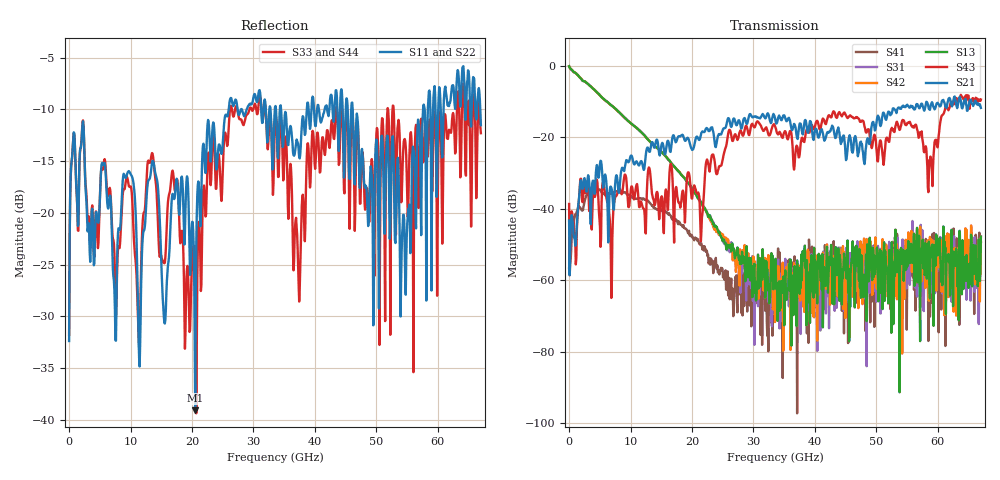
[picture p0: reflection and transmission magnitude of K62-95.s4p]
!Agilent Technologies,N5247A,US50470101,A.10.25.02
!Agilent N5247A: A.10.25.02
!Date: Tuesday, May 12, 2015 13:46:24
!Correction: Sdd11(Full 4 Port(1,2,3,4))
!Sdc11(Full 4 Port(1,2,3,4))
!Sdd12(Full 4 Port(1,2,3,4))
!Sdc12(Full 4 Port(1,2,3,4))
!Scd11(Full 4 Port(1,2,3,4))
!Scc11(Full 4 Port(1,2,3,4))
!Scd12(Full 4 Port(1,2,3,4))
!Scc12(Full 4 Port(1,2,3,4))
!Sdd21(Full 4 Port(1,2,3,4))
!Sdc21(Full 4 Port(1,2,3,4))
!Sdd22(Full 4 Port(1,2,3,4))
!Sdc22(Full 4 Port(1,2,3,4))
!Scd21(Full 4 Port(1,2,3,4))
!Scc21(Full 4 Port(1,2,3,4))
!Scd22(Full 4 Port(1,2,3,4))
!Scc22(Full 4 Port(1,2,3,4))
!Balanced Topology: BBAL
!S4P File: Measurements: <Sdd11,Sdc11,Sdd12,Sdc12>,
!<Scd11,Scc11,Scd12,Scc12>,
!<Sdd21,Sdc21,Sdd22,Sdc22>,
!<Scd21,Scc21,Scd22,Scc22>:
# Hz S  dB  R 50
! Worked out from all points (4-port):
!   801 points, 10 MHz to 67 GHz, reference 50 ohm
!   strongest paths, dB at 10 MHz, 16.76 GHz, 33.51 GHz, 50.25 GHz, 67 GHz:
!     S21: -43.3, -20.7, -14.6, -13.9, -11.8
!     S43: -38.6, -29.4, -16.9, -26.7, -9.4
!     S13: -0.1, -27.5, -55.4, -61.9, -47.8
!     S42: -0.1, -27.5, -71.7, -51.7, -49.3
!     S31: -0.1, -27.5, -60.2, -50.4, -49.3
!     S41: -56.7, -42.4, -57.1, -55.7, -47.8
!   lowest |S11| = -39.1 dB at 20.53 GHz (marker M1), VSWR 1.02, Z = 51 - j0.416 ohm
!   |S11| at or under -10 dB: start of sweep to 25.98 GHz; 34.49 GHz to 38.68 GHz (4.195 GHz wide, 11.5 % of centre); 46.15 GHz to 57.6 GHz (11.45 GHz wide, 22.1 % of centre)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
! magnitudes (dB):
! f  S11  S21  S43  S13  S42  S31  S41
! 10 MHz  -32.4  -43.3  -38.6  -0.1  -0.1  -0.1  -56.7
! 4.699 GHz  -20.9  -29.9  -35.1  -7.7  -7.7  -7.7  -34.9
! 6.876 GHz  -20.0  -34.1  -64.9  -11.0  -11.1  -11.1  -35.8
! 20.53 GHz  -39.1  -21.0  -34.2  -35.6  -35.7  -35.6  -48.0
! 34.34 GHz  -9.7  -14.5  -18.7  -61.6  -62.5  -66.8  -69.4
! 58.71 GHz  -8.6  -12.3  -26.7  -65.1  -47.9  -62.1  -70.1
! 67 GHz  -11.5  -11.8  -9.4  -47.8  -49.3  -49.3  -47.8
